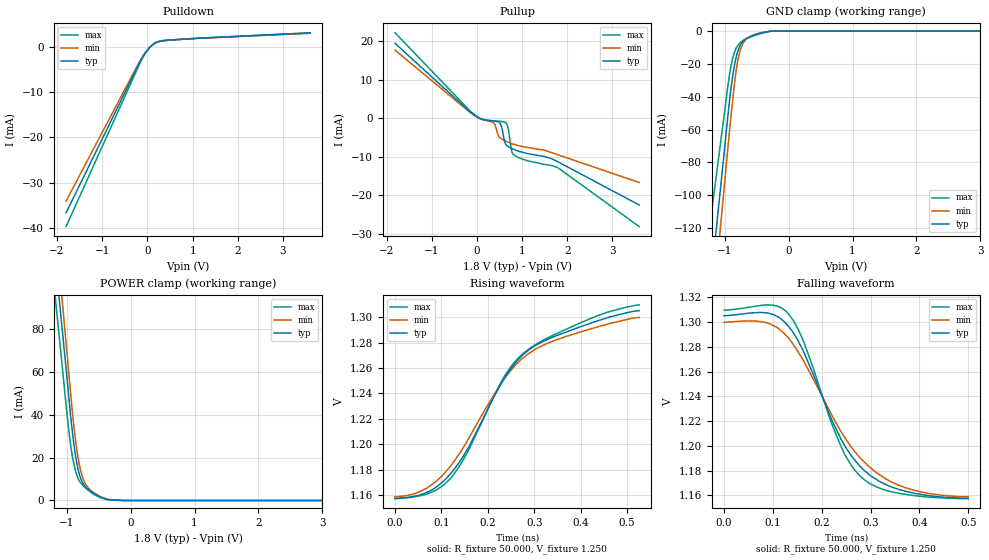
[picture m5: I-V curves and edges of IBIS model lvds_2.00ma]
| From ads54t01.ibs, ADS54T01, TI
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[Model]   lvds_2.00ma
Model_type 3-state
Vref=1.250E+00
Rref=5.000E+01
Cref=0.000E+00
Vmeas=1.250E+00
C_comp   7.860E-13   7.790E-13   7.930E-13
[Voltage Range]   1.800E+00   1.650E+00   1.950E+00
[POWER Clamp Reference]   1.800E+00   1.650E+00   1.950E+00
[GND Clamp Reference]   0.000E+00   0.000E+00   0.000E+00
[Pullup Reference]   1.800E+00   1.650E+00   1.950E+00
[Pulldown Reference]   0.000E+00   0.000E+00   0.000E+00
[Temperature Range]   25   85   -40
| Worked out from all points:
|   slope of the pulldown table from 0 to 0.27 V, typ, clamps not added: 137 ohm
|   slope of the pullup table from 0 to 0.27 V, typ, clamps not added: 286 ohm
|   GND clamp passes 1 mA (typ) near -0.41 V on its own axis
|   POWER clamp passes 1 mA (typ) near -0.41 V on its own axis
|   rising waveform, R_fixture 50.000, V_fixture 1.250: 20-80 % time 153ps typ, 161ps min, 159ps max; typ from 1.16 V to 1.3 V
|   falling waveform, R_fixture 50.000, V_fixture 1.250: 20-80 % time 107ps typ, 128ps min, 87.5ps max; typ from 1.3 V to 1.16 V
[GND Clamp]
-1.8V     -374.4mA   -423.5mA   -288.4mA
-1.02V    -78.69mA   -100.5mA   -54.92mA
-920mV    -41.17mA   -59.34mA   -25.51mA
-860mV    -23.88mA   -36.88mA   -14.48mA
-820mV    -15.94mA   -23.97mA   -10.43mA
-780mV    -10.76mA   -15.27mA   -8.038mA
-740mV    -7.589mA   -9.923mA   -6.562mA
-700mV    -5.657mA   -6.755mA   -5.499mA
-640mV    -4.069mA   -4.329mA   -4.359mA
-460mV    -1.489mA   -1.354mA   -1.806mA
-220mV    -4.201uA   -14.01uA   -11.29uA
3.6V      0A         0A         0A
[Power Clamp]
-1.8V     302.8mA    334.3mA    279.3mA
-1.76V    290.6mA    320.1mA    266.6mA
-1.06V    77.25mA    90.47mA    60.21mA
-940mV    40.5mA     50.88mA    26.54mA
-880mV    24.97mA    33.1mA     16.1mA
-820mV    14.43mA    19.78mA    10.24mA
-780mV    10.23mA    13.83mA    8.195mA
-720mV    6.913mA    8.542mA    6.262mA
-580mV    3.451mA    3.702mA    2.982mA
-360mV    441.4uA    538.8uA    356.5uA
-140mV    0A         9.789uA    18.55uA
3.6V      0A         0A         0A
[Pullup]
-1.82V    19.46mA    17.7mA     22.21mA
-140mV    1.529mA    1.362mA    1.727mA
60mV      -47.21uA   -99.84uA   23.69uA
360mV     -747.5uA   -1.024mA   -685.1uA
500mV     -1.146mA   -4.992mA   -814.3uA
560mV     -2.992mA   -5.485mA   -873.7uA
620mV     -6.397mA   -5.859mA   -1.028mA
680mV     -7.306mA   -6.197mA   -2.119mA
760mV     -7.802mA   -6.575mA   -8.093mA
800mV     -8.021mA   -6.737mA   -9.421mA
1.78V     -11.25mA   -9.45mA    -12.75mA
3.6V      -22.57mA   -16.72mA   -28.19mA
[Pulldown]
-1.8V     -36.69mA   -34.09mA   -39.71mA
-180mV    -3.673mA   -3.423mA   -3.971mA
-80mV     -1.887mA   -1.78mA    -2.015mA
40mV      -298uA     -308.1uA   -272.6uA
160mV     727uA      672.5uA    790.9uA
320mV     1.262mA    1.249mA    1.257mA
520mV     1.452mA    1.46mA     1.422mA
3.6V      3.011mA    2.915mA    3.027mA
[Rising Waveform]
R_fixture = 50.000
V_fixture = 1.250
V_fixture_min = 1.250
V_fixture_max = 1.250
|  time   V(typ)   V(min)   V(max)
0s        1.158V     1.159V     1.157V
68ps      1.162V     1.165V     1.161V
120ps     1.177V     1.183V     1.173V
156ps     1.196V     1.203V     1.194V
232ps     1.25V      1.25V      1.251V
256ps     1.263V     1.261V     1.264V
288ps     1.274V     1.271V     1.275V
338ps     1.284V     1.281V     1.285V
436ps     1.297V     1.292V     1.301V
526ps     1.305V     1.3V       1.31V
[Falling Waveform]
R_fixture = 50.000
V_fixture = 1.250
V_fixture_min = 1.250
V_fixture_max = 1.250
|  time   V(typ)   V(min)   V(max)
0s        1.305V     1.3V       1.31V
88ps      1.307V     1.299V     1.314V
116ps     1.303V     1.293V     1.312V
134ps     1.296V     1.286V     1.306V
164ps     1.275V     1.268V     1.283V
240ps     1.205V     1.211V     1.199V
264ps     1.19V      1.197V     1.182V
288ps     1.18V      1.186V     1.172V
372ps     1.163V     1.166V     1.161V
500ps     1.158V     1.159V     1.157V
[Ramp]
dV/dt_r   8.8560E-02/1.5250E-10   8.4600E-02/1.6090E-10   9.1500E-02/1.5850E-10
dV/dt_f   8.8560E-02/1.0691E-10   8.4600E-02/1.2806E-10   9.1500E-02/8.7078E-11
R_load = 50
